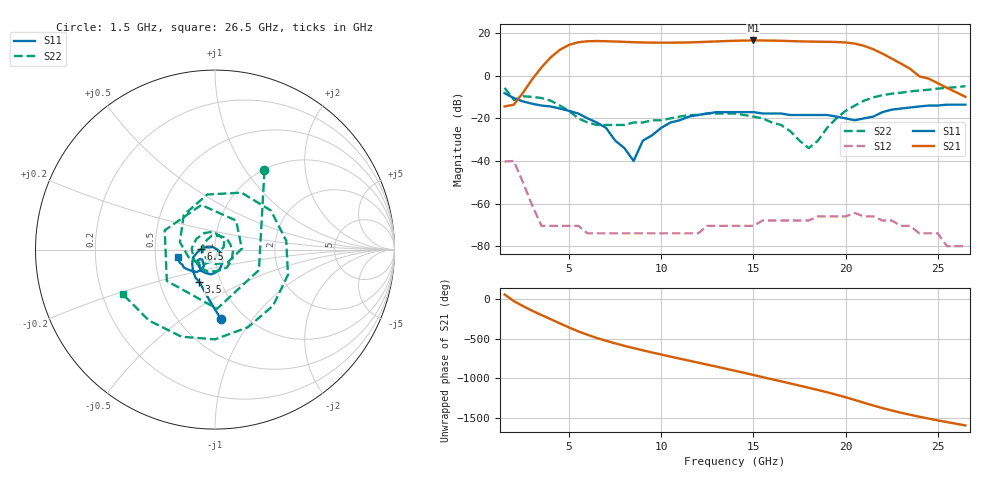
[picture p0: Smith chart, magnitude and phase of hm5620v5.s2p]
!  HMMC-5620
!  S-PARAMETERS  at  Vdd = 5V;  Idd = 100mA.  LAST UPDATED  02-07-97
#  GHZ  S  MA  R  50
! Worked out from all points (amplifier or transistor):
!   51 points, 1.5 GHz to 26.5 GHz, reference 50 ohm
!   highest |S21| = 16.6 dB at 15 GHz (marker M1)
!   |S21| within 3 dB of that: 4.795 GHz to 21.15 GHz (16.35 GHz wide, 126 % of centre)
!   unconditionally stable (mu >= 1): start of sweep to end of sweep
!   at 5.5 GHz: K = 265.05, MAG = 15.9 dB, |S12| = -70.5 dB
!   at 14 GHz: K = 242.65, MAG = 16.6 dB, |S12| = -70.5 dB
!   at 26.5 GHz: K = 10083.18, MAG = -8.0 dB, |S12| = -80.0 dB
!   S11 on the Smith chart (normalised r, x): 1.5 GHz: 0.78, -0.72; 3.5 GHz: 0.79, -0.30; 6.5 GHz: 0.85, +0.00; 26.5 GHz: 0.66, -0.06
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1.5  0.39 -85.0  0.19 58.0  0.0097 -21.0  0.52 58.0
3.5  0.2 -116.0  1.57 159.0  0.0003 142.0  0.3 159.0
4.5  0.17 -136.0  4.08 54.0  0.0003 168.0  0.2 54.0
5  0.15 -148.0  5.32 2.0  0.0003 144.0  0.15 2.0
6  0.1 -171.0  6.46 -90.0  0.0002 86.0  0.08 -90.0
6.5  0.08 179.0  6.54 -130.0  0.0002 55.0  0.07 -130.0
7.5  0.03 156.0  6.36 162.0  0.0002 -5.0  0.07 162.0
8.5  0.01 13.0  6.13 102.0  0.0002 -51.0  0.08 102.0
10  0.06 -48.0  5.97 21.0  0.0002 -98.0  0.09 21.0
11  0.09 -66.0  6.01 -31.0  0.0002 -122.0  0.11 -31.0
12  0.12 -83.0  6.16 -81.0  0.0002 -145.0  0.12 -81.0
13  0.14 -99.0  6.4 -132.0  0.0003 -167.0  0.13 -132.0
14  0.14 -114.0  6.62 176.0  0.0003 170.0  0.13 176.0
15  0.14 -125.0  6.74 123.0  0.0003 145.0  0.11 123.0
16  0.13 -132.0  6.69 69.0  0.0004 119.0  0.08 69.0
17  0.12 -135.0  6.52 16.0  0.0004 92.0  0.05 16.0
18.5  0.12 -143.0  6.3 -66.0  0.0005 49.0  0.03 -66.0
19  0.12 -146.0  6.26 -95.0  0.0005 32.0  0.06 -95.0
20  0.1 -148.0  6.05 -158.0  0.0005 -6.0  0.15 -158.0
21  0.1 -131.0  5.04 132.0  0.0005 -52.0  0.26 132.0
22.5  0.16 -129.0  2.54 35.0  0.0004 -116.0  0.38 35.0
26.5  0.21 -169.0  0.32 -154.0  0.0001 139.0  0.57 -154.0
